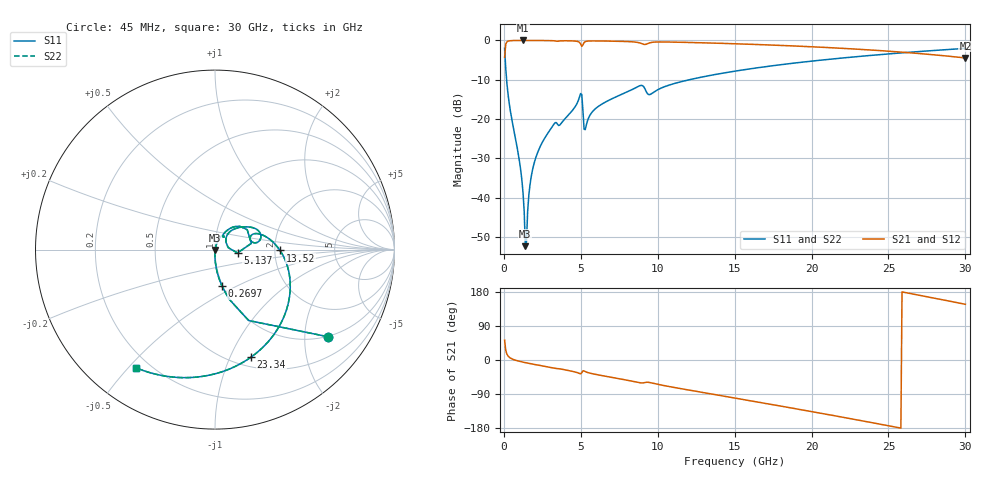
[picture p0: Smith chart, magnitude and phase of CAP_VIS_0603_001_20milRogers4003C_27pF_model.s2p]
! S-parameter model data by Modelithics Inc.  support@modelithics.com  813-866-6335  Tampa FL USA
! S-Parameter data specifications:
! Substrate: 20-mil Rogers 4003C, substrate thickness, H=0.508mm, Dielectric constant, Er=3.75
! PCB Mounting Pad Footprint: Pad width, PadW=0.90mm , Pad length, PadL=1.00mm , Pad gap, PadG (edge-to-edge)=1.00mm , Reference planes=3.0mm apart
! Created Wed Nov 18 13:27:48 2015
# hz S ma R 50
! 2 Port Network Data from SP1.SP block
! freq  magS11  angS11  magS21  angS21  magS12  angS12  magS22  angS22
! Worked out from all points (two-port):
!   401 points, 45 MHz to 30 GHz, reference 50 ohm
!   highest |S21| = -0.01 dB at 1.243 GHz (marker M1); lowest = -4.5 dB at 30 GHz (marker M2)
!   |S21| within 3 dB of the highest: 73.79 MHz to 25.96 GHz (25.89 GHz wide, 199 % of centre)
!   lowest |S11| = -52.3 dB at 1.393 GHz (marker M3), VSWR 1.00, Z = 50.1 - j0.213 ohm
!   |S11| at or under -10 dB: 176 MHz to 12.05 GHz (11.88 GHz wide, 194 % of centre)
!   |S22| runs from -52.3 to -2.0 dB; largest |S21 - S12| = 0
!   S11 on the Smith chart (normalised r, x): 45 MHz: 0.99, -2.59; 269.7 MHz: 0.99, -0.42; 5.137 GHz: 1.29, -0.05; 13.52 GHz: 2.14, -0.02; 23.34 GHz: 0.60, -1.20; 30 GHz: 0.15, -0.53
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4.5e7  0.7935 -37.7  0.6084 52.3  0.6084 52.3  0.7935 -37.7
2.696625e8  0.2055 -79.3  0.978 10.5  0.978 10.5  0.2055 -79.3
1.018538e9  0.02841 -91.1  0.9983 -3.5  0.9983 -3.5  0.02841 -91.1
1.2432e9  0.01152 -89.0  0.9985 -5.6  0.9985 -5.6  0.01152 -89.0
1.392975e9  0.002422 -61.6  0.9985 -6.9  0.9985 -6.9  0.002422 -61.6
1.54275e9  0.006706 69.1  0.9984 -8.2  0.9984 -8.2  0.006706 69.1
1.8423e9  0.02176 75.1  0.998 -10.6  0.998 -10.6  0.02176 75.1
2.4414e9  0.04829 72.5  0.9966 -15.1  0.9966 -15.1  0.04829 72.5
4.912688e9  0.1901 42.8  0.9439 -35.6  0.9439 -35.6  0.1901 42.8
5.062462e9  0.2053 9.8  0.8407 -33.7  0.8407 -33.7  0.2053 9.8
5.13735e9  0.127 -8.4  0.8793 -28.5  0.8793 -28.5  0.127 -8.4
5.362012e9  0.08479 44.0  0.9755 -31.8  0.9755 -31.8  0.08479 44.0
6.93465e9  0.1778 43.2  0.9789 -45.3  0.9789 -45.3  0.1778 43.2
8.806838e9  0.2642 23.2  0.9318 -59.8  0.9318 -59.8  0.2642 23.2
9.480825e9  0.2047 17.3  0.9322 -59.5  0.9322 -59.5  0.2047 17.3
1.007992e10  0.2404 21.8  0.9559 -64.9  0.9559 -64.9  0.2404 21.8
1.352475e10  0.3622 -0.8  0.9254 -89.9  0.9254 -89.9  0.3622 -0.8
1.50225e10  0.4067 -11.2  0.9067 -100.5  0.9067 -100.5  0.4067 -11.2
2.003996e10  0.5463 -47.0  0.8296 -136.4  0.8296 -136.4  0.5463 -47.0
2.333501e10  0.6316 -71.4  0.7661 -160.8  0.7661 -160.8  0.6316 -71.4
2.505742e10  0.6747 -84.5  0.7282 -174.0  0.7282 -174.0  0.6747 -84.5
3e10  0.7915 -123.6  0.5986 147.0  0.5986 147.0  0.7915 -123.6
